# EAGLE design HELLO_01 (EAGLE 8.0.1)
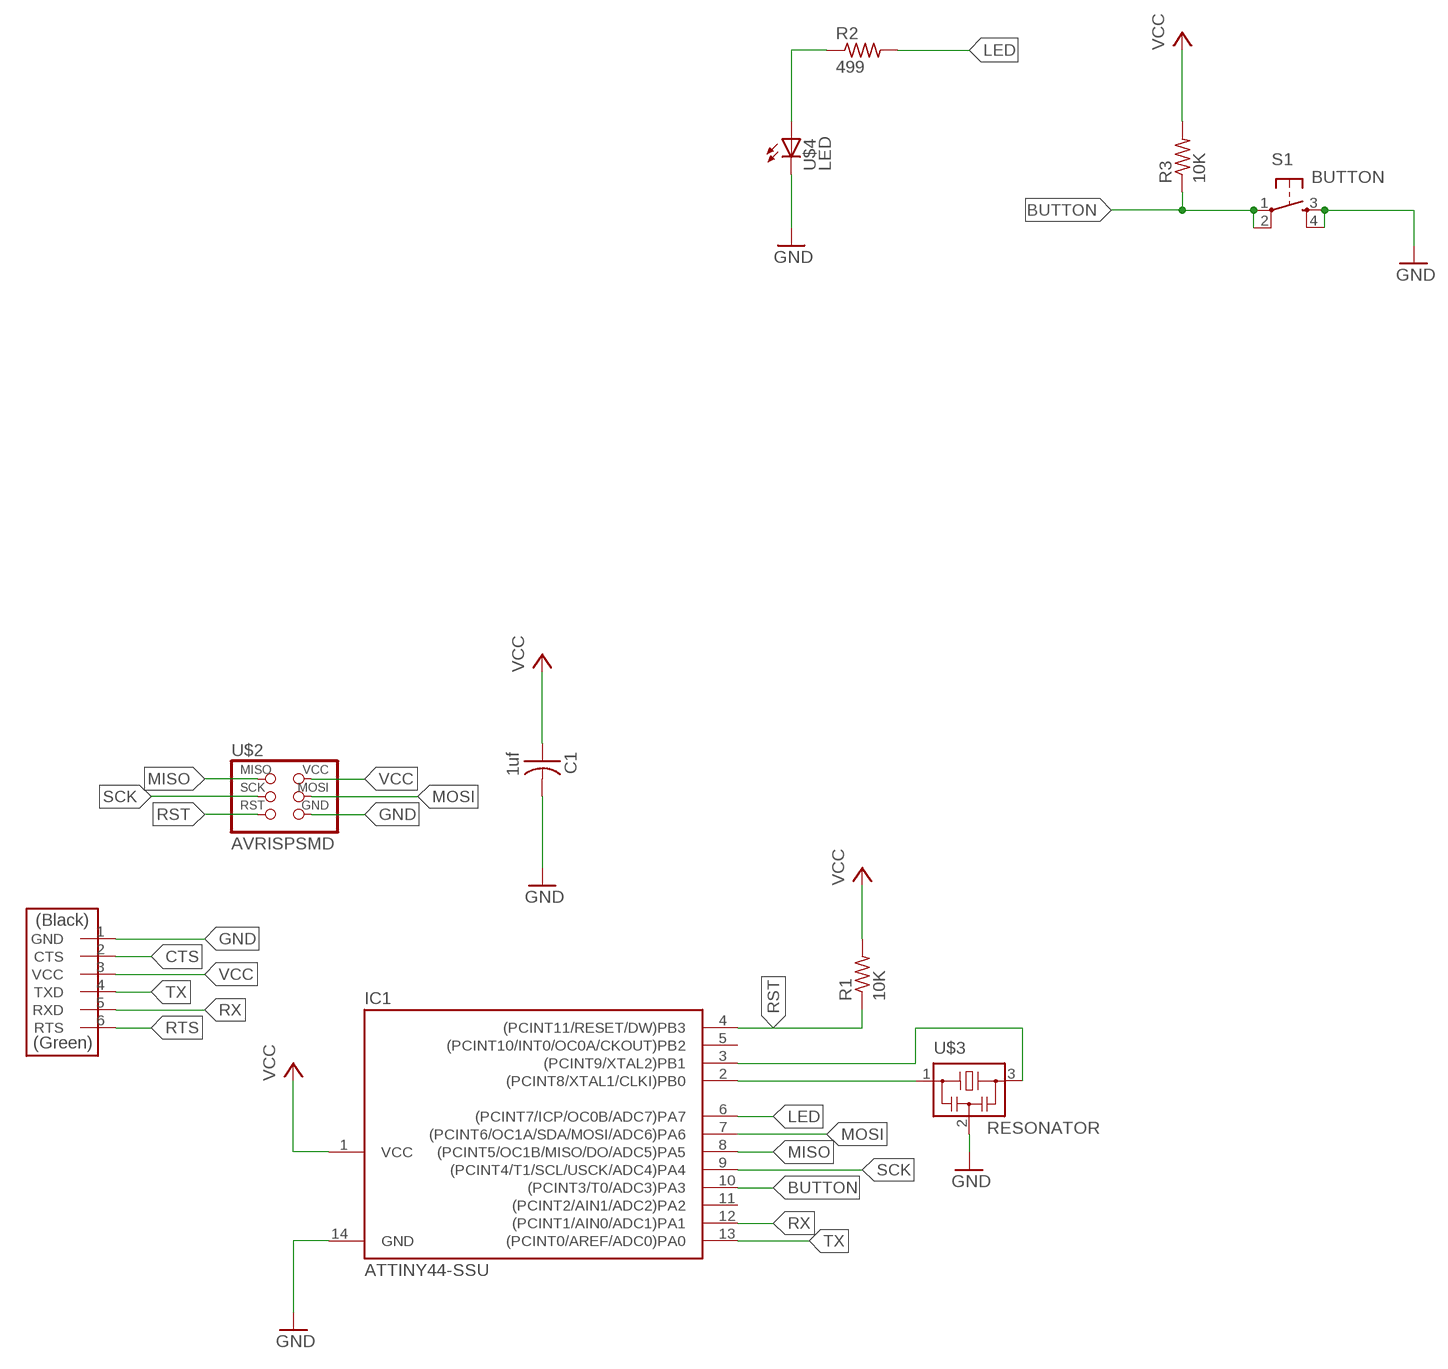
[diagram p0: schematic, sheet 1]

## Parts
C1  1uf  CAP-US1206FAB  [C1206FAB]
IC1  ATTINY44-SSU  [SOIC14]
R1  10K  RES-US1206FAB  [R1206FAB]
R2  499  RES-US1206FAB  [R1206FAB]
R3  10K  RES-US1206FAB  [R1206FAB]
S1  BUTTON  6MM_SWITCH6MM_SWITCH  [6MM_SWITCH]
U$1  FTDI-SMD-HEADER  [1X06SMD]
U$2  AVRISPSMD  [2X03SMD]
U$3  RESONATOR  [EFOBM]
U$4  LED  LEDFAB1206  [LED1206FAB]

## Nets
BUTTON: IC1.10((PCINT3/T0/ADC3)PA3) R3.1 S1.1(P) S1.2(P1)
CTS: U$1.2(CTS)
GND: C1.2 IC1.14(GND) S1.3(S) S1.4(S1) U$1.1(GND) U$2.6(GND) U$3.2 U$4.2(C)
LED: IC1.6((PCINT7/ICP/OC0B/ADC7)PA7) R2.2
MISO: IC1.8((PCINT5/OC1B/MISO/DO/ADC5)PA5) U$2.1(MISO)
MOSI: IC1.7((PCINT6/OC1A/SDA/MOSI/ADC6)PA6) U$2.4(MOSI)
N$25: IC1.2((PCINT8/XTAL1/CLKI)PB0) U$3.1
N$26: IC1.3((PCINT9/XTAL2)PB1) U$3.3
N$33: R2.1 U$4.1(A)
RST: IC1.4((PCINT11/RESET/DW)PB3) R1.1 U$2.5(RST)
RTS: U$1.6(RTS)
RX: IC1.12((PCINT1/AIN0/ADC1)PA1) U$1.5(RXD)
SCK: IC1.9((PCINT4/T1/SCL/USCK/ADC4)PA4) U$2.3(SCK)
TX: IC1.13((PCINT0/AREF/ADC0)PA0) U$1.4(TXD)
VCC: C1.1 IC1.1(VCC) R1.2 R3.2 U$1.3(VCC) U$2.2(VCC)
Unconnected: IC1.5((PCINT10/INT0/OC0A/CKOUT)PB2) IC1.11((PCINT2/AIN1/ADC2)PA2)

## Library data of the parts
C1 = fab:CAP-US
IC1 = fab:ATTINY44
R1-R3 = fab:RES-US: Resistor (US Symbol)
S1 = fab:6MM_SWITCH: OMRON SWITCH
U$1 = fab:FTDI-SMD-HEADER
U$2 = fab:AVRISP
U$3 = fab:RESONATOR
U$4 = fab:LED: LED

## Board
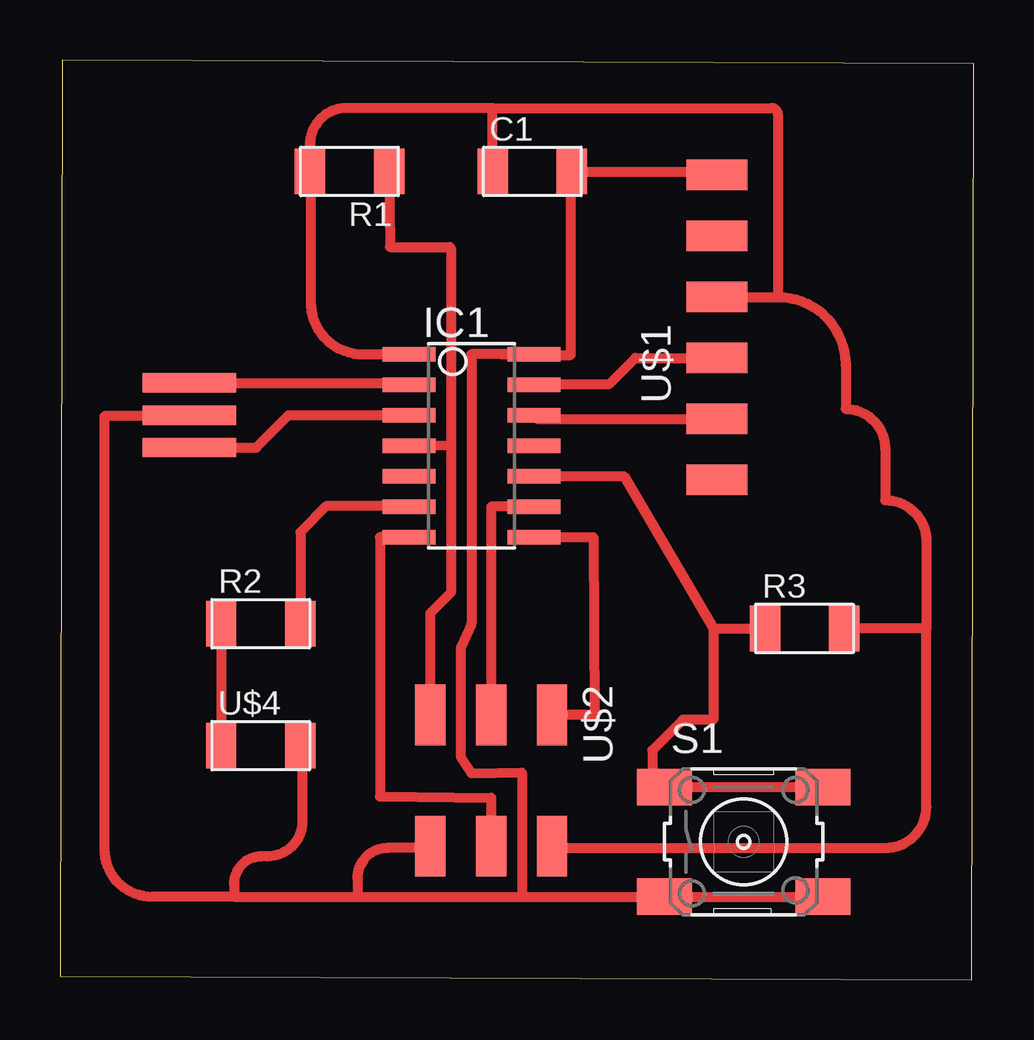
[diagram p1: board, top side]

Size 38.1 x 38.35 mm. Coordinates in mm from the lower left corner, seen from the top.
Outline: 0,0.15 38,0 38.1,38.2 0.1,38.35 0,0.15
Copper layers (1*16): Top 0.035mm / dielectric 1.5mm / Bottom 0.035mm
Design rules "default *": minimum track width 10mil, minimum drill 24mil, track to track 16mil, track to pad 16mil, pad to pad 16mil, via to via 16mil, smd to smd 16mil, copper to edge 40mil, drill to drill 8mil, minimum pad ring 10mil, minimum via ring 8mil, stop-mask expansion 4mil, vias tented up to drill 0mil, thermal gap 10mil

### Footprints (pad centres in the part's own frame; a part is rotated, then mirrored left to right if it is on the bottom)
C1206FAB = smd 1.27 x 1.905: 1 -1.651,0; 2 1.651,0
SOIC14 = smd 0.61 x 2.21: 1 -3.81,-2.603; 2 -2.54,-2.603; 3 -1.27,-2.603; 4 0,-2.603; 5 1.27,-2.603; 6 2.54,-2.603; 7 3.81,-2.603; 8 3.81,2.603; 9 2.54,2.603; 10 1.27,2.603; 11 0,2.603; 12 -1.27,2.603; 13 -2.54,2.603; 14 -3.81,2.603
R1206FAB = smd 1.27 x 1.905: 1 -1.651,0; 2 1.651,0
6MM_SWITCH = smd 2.286 x 1.524: 1 -3.302,2.286; 2 3.302,2.286; 3 -3.302,-2.286; 4 3.302,-2.286
1X06SMD = smd 2.54 x 1.27: 1 0,6.35; 2 0,3.81; 3 0,1.27; 4 0,-1.27; 5 0,-3.81; 6 0,-6.35
2X03SMD = smd 2.54 x 1.27: 1 -2.54,2.54; 2 2.92,2.54; 3 -2.54,0; 4 2.92,0; 5 -2.54,-2.54; 6 2.92,-2.54
EFOBM = smd 0.8 x 3.9: 1 -1.35,0; 2 0,0; 3 1.35,0
LED1206FAB = smd 1.27 x 1.905: 1 -1.651,0; 2 1.651,0

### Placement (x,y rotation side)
C1  19.69,33.7 0 top
IC1  17.15,22.27 270 top
R1  12.07,33.7 180 top
R2  8.37,14.85 0 top
R3  31.04,14.65 0 top
S1  28.5,5.76 0 top
U$1  27.38,27.2 0 top
U$2  17.97,8.5 270 top
U$3  5.39,23.54 270 top
U$4  8.37,9.77 0 top

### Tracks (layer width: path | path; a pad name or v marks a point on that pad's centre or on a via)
BUTTON
  Top 0.406: IC1.10 23.5,21 27.23,14.65 | 27.23,14.65 R3.1 | 27.23,14.65 27.23,10.84 25.96,10.84 24.69,9.57 24.69,8.55 S1.1 S1.2
GND
  Top 0.406: S1.3 24.94,3.22 | S1.3 S1.4 | 18.42,26.08 IC1.14 | IC1.14 17.15,26.08 17.15,14.85 16.7,13.85 16.7,9.3 17.15,8.62 19.25,8.65 19.25,3.47 | U$3.2 5.35,23.5 1.85,23.5 1.85,5.45 arc90 3.83,3.47 7.25,3.47 | 7.25,3.47 12.4,3.47 | 12.4,3.47 19.25,3.47 | 19.25,3.47 S1.3 | U$2.6 arc-90 15.35,5.5 13.65,5.5 arc90 12.4,4.25 12.4,3.47 | U$4.2 arc-90 10.1,9.69 10.1,6.6 arc-90 8.65,5.15 8.4,5.15 arc90 7.25,4 7.25,3.47 | U$1.1 27.38,33.7 C1.2 21.3,33.7 21.3,26.05 19.75,26.05 IC1.14
LED
  Top 0.406: IC1.6 14.53,19.75 11.1,19.75 10.02,18.67 R2.2
MISO
  Top 0.406: IC1.8 22.23,18.46 22.28,11.04 U$2.1
MOSI
  Top 0.406: IC1.7 13.34,18.46 13.34,7.65 17.97,7.6 U$2.4
N$25
  Top 0.406: U$3.1 14.47,24.89 IC1.2
N$26
  Top 0.406: U$3.3 8.18,22.19 9.53,23.54 IC1.3
N$33
  Top 0.406: R2.1 U$4.1
RST
  Top 0.406: R1.1 13.75,30.55 16.25,30.55 16.3,30.5 16.3,22.3 | IC1.4 16.3,22.3 | 16.3,22.3 16.3,16.15 15.43,15.28 U$2.5
RX
  Top 0.406: IC1.12 19.9,23.39 U$1.5
SCK
  Top 0.406: IC1.9 17.97,19.73 U$2.3
TX
  Top 0.406: IC1.13 19.79,24.85 22.9,24.85 23.98,25.93 U$1.4
VCC
  Top 0.406: 29.92,28.47 29.92,36.09 arc90 29.66,36.35 18.04,36.35 | 10.8,34.08 R1.2 | U$1.3 29.92,28.47 | 36.12,14.65 R3.2 | 18.04,36.35 11.95,36.35 arc90 10.42,34.82 R1.2 | C1.1 18.04,36.35 | R1.2 arc-90 10.45,33.67 10.45,28.25 arc90 12.62,26.08 IC1.1 | U$2.2 arc90 20.59,5.5 34.4,5.5 arc90 36.12,7.22 36.12,14.65 | 29.92,28.47 arc-90 32.75,25.64 32.75,23.8 arc-90 34.4,22.15 34.4,20 arc-90 36.12,18.28 36.12,14.65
